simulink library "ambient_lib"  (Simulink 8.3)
settings: Solver=ode45  StartTime=0.0  StopTime=10.0  RelTol=1e-3
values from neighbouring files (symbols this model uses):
  ambient = class_REVS_ambient    [ambient_param.m]    (also in REVS_run_preproc.m)
undefined symbols (not defined in the file or in its folder): drive_cycle
libraries: general_lib x1

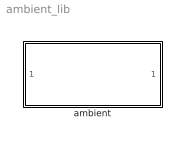
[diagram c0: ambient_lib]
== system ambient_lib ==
  ambient : Subsystem

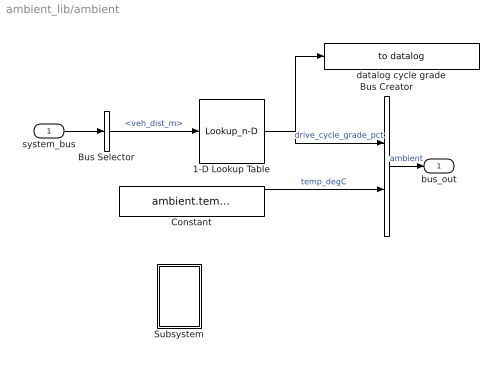
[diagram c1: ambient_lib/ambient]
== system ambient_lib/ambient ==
  system_bus : Inport
  1-D Lookup Table : Lookup_n-D  NumberOfTableDimensions=1  BreakpointsForDimension1=drive_cycle.grade_dist_m  IndexSearchMethod=Linear search  BeginIndexSearchUsingPreviousIndexResult=on  Table=drive_cycle.grade_pct  ExtrapMethod=Clip  UseLastTableValue=on  RndMeth=Simplest
  Bus Creator : BusCreator  Inputs=2
  Bus Selector : BusSelector  OutputSignals=signal4.veh_dist_m
  Constant : Constant  Value=ambient.temperature_degC
  Subsystem : Subsystem
  datalog cycle grade : general_lib/to datalog  VarName=drive_cycle_grade_pct  WorkspaceName=datalog__drive_cycle_grade_pct  VerboseLevel=1  VerboseSignal=REVS.verbose
  bus_out : Outport
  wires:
  Bus Selector/1 -> 1-D Lookup Table/1  "<veh_dist_m>"
  system_bus/1 -> Bus Selector/1
  Bus Creator/1 -> bus_out/1  "ambient"
  1-D Lookup Table/1 -> Bus Creator/1, datalog cycle grade/1  "drive_cycle_grade_pct"
  Constant/1 -> Bus Creator/2  "temp_degC"

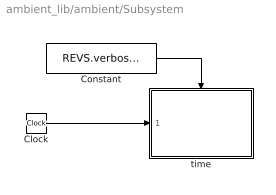
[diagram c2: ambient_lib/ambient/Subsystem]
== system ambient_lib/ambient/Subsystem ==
  Clock : Clock
  Constant : Constant  Value=REVS.verbose >= 0
  time : Subsystem
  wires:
  Clock/1 -> time/1("time ")
  Constant/1 -> time/Enable

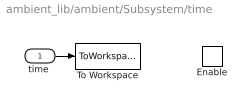
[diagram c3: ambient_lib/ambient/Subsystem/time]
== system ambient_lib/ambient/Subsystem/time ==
  "time " : Inport
  Enable : EnablePort
  To Workspace : ToWorkspace  VariableName=time  SampleTime=-1
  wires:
  "time "/1 -> To Workspace/1
